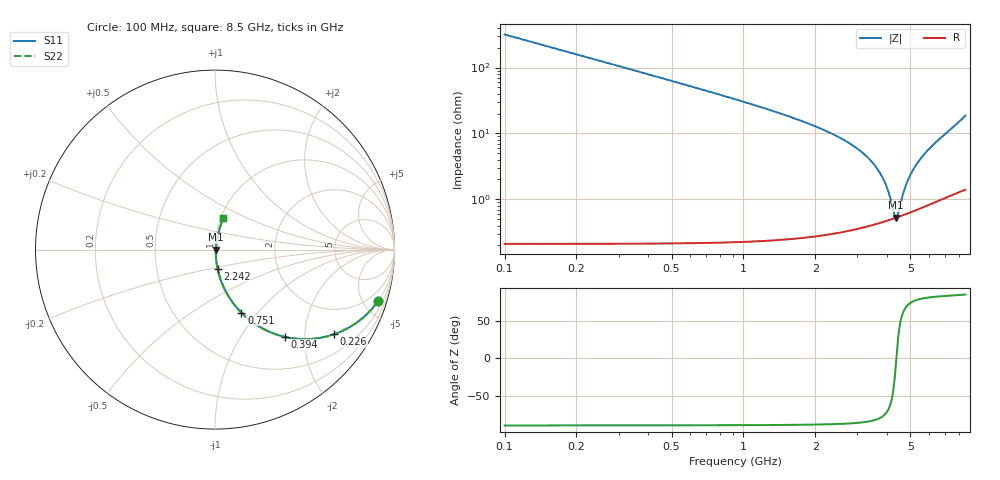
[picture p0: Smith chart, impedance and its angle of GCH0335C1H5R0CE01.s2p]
!Murata Part Number: GCH0335C1H5R0CE01
!These Parameters are Measured in Series Mode Connection
!Data Generated on Mar 13, 2026
!  o--ll--o
!Port1  Port2
!  o------o
!Operation Temp=25[degC], DC Bias Voltage=0[V]
!Freq. Start=100[MHz] Stop=9[GHz] 401[Steps]
# Hz S RI R 50
!Freq.(Hz) S11(Real) S11(Imag) S21(Real) S21(Imag) S12(Real) S12(Imag) S22(Real) S22(Imag)
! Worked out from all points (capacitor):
!   401 points, 100 MHz to 8.5 GHz, reference 50 ohm
!   read as one part in series: C = 5 pF near 142 MHz
!   lowest |Z| = 527 mohm at 4.363 GHz (marker M1)
!   series resonance near 4.368 GHz, so ESL is about 270 pH
!   S11 on the Smith chart (normalised r, x): 100 MHz: 1.00, -6.36; 226 MHz: 1.00, -2.81; 394 MHz: 1.00, -1.60; 751 MHz: 1.00, -0.82; 2.242 GHz: 1.01, -0.21; 8.5 GHz: 1.03, +0.37
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1e8  0.9099 -0.2859  0.0901 0.2859  0.0901 0.2859  0.9099 -0.2859
2.26e8  0.6635 -0.4718  0.3365 0.4718  0.3365 0.4718  0.6635 -0.4718
3.94e8  0.3917 -0.4868  0.6083 0.4868  0.6083 0.4868  0.3917 -0.4868
5.62e8  0.2382 -0.4241  0.7618 0.4241  0.7618 0.4241  0.2382 -0.4241
7.51e8  0.1467 -0.3512  0.8533 0.3512  0.8533 0.3512  0.1467 -0.3512
1.045e9  0.0787 -0.2653  0.9213 0.2653  0.9213 0.2653  0.0787 -0.2653
1.507e9  0.0364 -0.1808  0.9636 0.1808  0.9636 0.1808  0.0364 -0.1808
2.242e9  0.0141 -0.1053  0.9859 0.1053  0.9859 0.1053  0.0141 -0.1053
2.914e9  0.00739 -0.0625  0.9926 0.0625  0.9926 0.0625  0.00739 -0.0625
3.418e9  0.00542 -0.0379  0.9946 0.0379  0.9946 0.0379  0.00542 -0.0379
3.775e9  0.00493 -0.0227  0.9951 0.0227  0.9951 0.0227  0.00493 -0.0227
4.027e9  0.00491 -0.0128  0.9951 0.0128  0.9951 0.0128  0.00491 -0.0128
4.3e9  0.00515 -0.0025  0.9949 0.0025  0.9949 0.0025  0.00515 -0.0025
4.363e9  0.00523 -0.000185  0.9948 0.000185  0.9948 0.000185  0.00523 -0.000185
4.447e9  0.00537 0.00286  0.9946 -0.00286  0.9946 -0.00286  0.00537 0.00286
4.72e9  0.00596 0.0126  0.994 -0.0126  0.994 -0.0126  0.00596 0.0126
4.93e9  0.00655 0.0199  0.9934 -0.0199  0.9934 -0.0199  0.00655 0.0199
5.266e9  0.00775 0.0315  0.9922 -0.0315  0.9922 -0.0315  0.00775 0.0315
5.707e9  0.0098 0.0467  0.9902 -0.0467  0.9902 -0.0467  0.0098 0.0467
6.295e9  0.0135 0.0675  0.9865 -0.0675  0.9865 -0.0675  0.0135 0.0675
7.114e9  0.0208 0.0997  0.9792 -0.0997  0.9792 -0.0997  0.0208 0.0997
8.5e9  0.0461 0.1757  0.9539 -0.1757  0.9539 -0.1757  0.0461 0.1757
